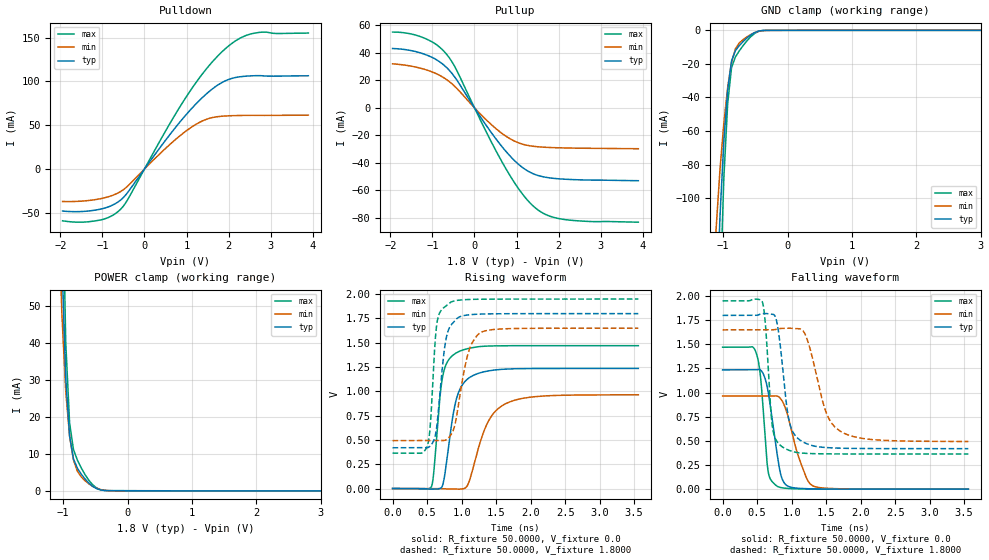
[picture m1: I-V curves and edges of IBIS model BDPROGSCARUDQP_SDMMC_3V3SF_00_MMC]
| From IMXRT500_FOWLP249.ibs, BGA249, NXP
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[Model] BDPROGSCARUDQP_SDMMC_3V3SF_00_MMC
|   Model BDPROGSCARUDQP_SDMMC_3V3SF_00_MMC
| This model was characterised for following simulation conditions:
| External (pad) voltage:
|   - Typ: 1.8V,   - Min: 1.65V,   - Max: 1.95V
| Library cells for typ/min/max conditions are connected as defined below:
|  IO - External Pad
|  A - Core Input
|  EN - Output Buffer Enable
|  ASRCN3V3[0] - REFH3V3
|  ASRCN3V3[1] - REFH3V3
|  ASRCN3V3[2] - REFH3V3
|  ASRCN3V3[3] - REFH3V3
|  ASRCP3V3[0] - REFL3V3
|  ASRCP3V3[1] - REFL3V3
|  ASRCP3V3[2] - REFL3V3
|  ASRCP3V3[3] - REFL3V3
|  IOGC - NC
|  PDRV - gnd
|  PSW - gnd
|  REFH3V3 - REFH3V3
|  REFL3V3 - REFL3V3
|  ZI - NC
|  gnd - gnd
|  gnde - gnde
|  vdd - vdd
|  vdde3v3 - vdde3v3
| All other pins connected to ground
Model_type I/O
Polarity   Non-Inverting
Enable   Active-Low
Vinl =   0.5775V
Vinh =   1.2675V
Vmeas =  0.9000V
Cref =   30.0000pF
Rref =   1.0000M
Vref =   1.8000V
C_comp   2.2202pF   2.2062pF   2.2431pF
|C_comp_pullup   1.1644pF   1.1332pF   1.1986pF
|C_comp_pulldown   0.0F   0.0F   0.0F
[Model Spec]
| variable   typ   min   max
Vinh   1.1700V   1.0725V   1.2675V
Vinl   0.6300V   0.5775V   0.6825V
|[Receiver Thresholds]
[Temperature Range]   25.0000   0.1050k   -20.0000
[Voltage Range]   1.8000V   1.6500V   1.9500V
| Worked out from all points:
|   slope of the pulldown table from 0 to 0.27 V, typ, clamps not added: 15.1 ohm
|   slope of the pullup table from 0 to 0.27 V, typ, clamps not added: 21.9 ohm
|   GND clamp passes 1 mA (typ) near -0.49 V on its own axis
|   POWER clamp passes 1 mA (typ) near -0.52 V on its own axis
|   rising waveform, R_fixture 50.0000, V_fixture 0.0: 20-80 % time 178ps typ, 301ps min, 120ps max; typ from 0 V to 1.24 V
|   rising waveform, R_fixture 50.0000, V_fixture 1.8000: 20-80 % time 121ps typ, 183ps min, 81.3ps max; typ from 0.42 V to 1.8 V
|   falling waveform, R_fixture 50.0000, V_fixture 0.0: 20-80 % time 151ps typ, 232ps min, 93.7ps max; typ from 1.24 V to 0 V
|   falling waveform, R_fixture 50.0000, V_fixture 1.8000: 20-80 % time 138ps typ, 264ps min, 86.9ps max; typ from 1.8 V to 0.42 V
[Pulldown]
|Voltage   I(typ)   I(min)   I(max)
-1.95V    -47.99mA   -37.12mA   -59.11mA
-1.05V    -45.86mA   -33.95mA   -58.21mA
-810mV    -42.31mA   -30.95mA   -54.25mA
-570mV    -35.53mA   -25.76mA   -46.04mA
-390mV    -26.13mA   -19.07mA   -34.15mA
510mV     33.34mA    23.88mA    44.03mA
1.11V     68.35mA    47.41mA    90.64mA
1.65V     92.58mA    59mA       124.1mA
2.07V     103.2mA    60.79mA    142.9mA
2.37V     105.7mA    61.13mA    151.4mA
2.67V     106.5mA    61.18mA    155.4mA
3.9V      106.4mA    61.45mA    155.1mA
[Pullup]
|Voltage   I(typ)   I(min)   I(max)
-1.95V    43.07mA    31.94mA    55mA
-1.2V     39.02mA    28.05mA    50.71mA
-900mV    34.81mA    24.65mA    45.75mA
-660mV    29.15mA    20.42mA    38.73mA
-420mV    20.14mA    14.1mA     27.04mA
240mV     -11.02mA   -7.543mA   -15.06mA
720mV     -30.63mA   -20.03mA   -42.78mA
1.14V     -43.3mA    -26.38mA   -62.56mA
1.5V      -49.04mA   -28.29mA   -73.94mA
1.8V      -50.95mA   -28.84mA   -78.8mA
2.16V     -51.88mA   -29.16mA   -81.21mA
3.9V      -52.96mA   -29.72mA   -83.09mA
[GND_clamp]
|Voltage   I(typ)   I(min)   I(max)
-1.95V    -1.765A    -1.022A    -2.885A
-1.11V    -175mA     -118.7mA   -274.2mA
-1.05V    -111.7mA   -83.43mA   -161.8mA
-990mV    -66.62mA   -55.67mA   -88.75mA
-930mV    -35.53mA   -34.14mA   -43.79mA
-870mV    -18.33mA   -19.05mA   -22.29mA
-810mV    -12.12mA   -11.08mA   -15.87mA
-750mV    -9.12mA    -7.575mA   -12.28mA
-570mV    -2.717mA   -2.477mA   -3.751mA
-450mV    -466.5uA   -625uA     -610.9uA
-330mV    -31.46uA   -57.07uA   -36.76uA
3.9V      0A         0A         0A
[POWER_clamp]
|Voltage   I(typ)   I(min)   I(max)
-1.95V    1.71A      976mA      2.836A
-1.08V    122.1mA    81.01mA    201.9mA
-1.02V    63.03mA    48mA       94.76mA
-960mV    30.4mA     27.02mA    40.25mA
-900mV    14.88mA    14.82mA    18.42mA
-840mV    8.668mA    8.369mA    11.21mA
-780mV    6.192mA    5.372mA    8.379mA
-720mV    4.573mA    3.84mA     6.25mA
-600mV    2.107mA    1.918mA    2.859mA
-480mV    625.6uA    714.7uA    800.1uA
-300mV    67.29uA    79.42uA    85.49uA
3.9V      0A         0A         0A
[Ramp]
| variable   typ   min   max
dV/dt_r  0.7412/0.1778n   0.5784/0.3008n   0.8818/0.1204n
dV/dt_f  0.8278/0.1380n   0.6934/0.2640n   0.9510/86.9648p
R_load = 50.0000
[Rising Waveform]
R_fixture= 50.0000
V_fixture= 0.0
V_fixture_min= 0.0
V_fixture_max= 0.0
|time   V(typ)   V(min)   V(max)
0s        117.6uV    109.5uV    139.1uV
562.4ps   -4.931mV   122.9uV    18.16mV
594.7ps   -4.277mV   173.7uV    152mV
677.9ps   -839.1uV   104.5uV    879.8mV
722.4ps   28.57mV    -1.56mV    1.139V
918ps     903.5mV    -5.529mV   1.394V
1.081ns   1.124V     27.34mV    1.438V
1.376ns   1.209V     676.5mV    1.466V
1.642ns   1.229V     874.3mV    1.469V
3.56ns    1.235V     964mV      1.47V
[Rising Waveform]
R_fixture= 50.0000
V_fixture= 1.8000
V_fixture_min= 1.6500
V_fixture_max= 1.9500
|time   V(typ)   V(min)   V(max)
0s        419.6mV    493.2mV    364.4mV
498.5ps   419.9mV    493.2mV    429.5mV
543.4ps   436.1mV    493.2mV    625mV
614.7ps   533mV      493.3mV    1.496V
647.5ps   681.8mV    493.2mV    1.722V
753.3ps   1.446V     495.5mV    1.868V
838.5ps   1.672V     545.1mV    1.915V
1.093ns   1.786V     1.388V     1.945V
1.264ns   1.795V     1.6V       1.948V
3.56ns    1.799V     1.649V     1.949V
[Falling Waveform]
R_fixture= 50.0000
V_fixture= 0.0
V_fixture_min= 0.0
V_fixture_max= 0.0
|time   V(typ)   V(min)   V(max)
0s        1.235V     964mV      1.47V
479.1ps   1.236V     964.3mV    1.426V
549.2ps   1.234V     964.2mV    1.168V
660.6ps   1.008V     964mV      181.4mV
790.5ps   364mV      964.1mV    30.51mV
847.8ps   138.2mV    931.1mV    16.13mV
916ps     45.91mV    827.4mV    9.318mV
1.116ns   8.351mV    304mV      2.793mV
1.315ns   3.043mV    32.47mV    1.081mV
3.56ns    124.6uV    222.5uV    139.7uV
[Falling Waveform]
R_fixture= 50.0000
V_fixture= 1.8000
V_fixture_min= 1.6500
V_fixture_max= 1.9500
|time   V(typ)   V(min)   V(max)
0s        1.799V     1.649V     1.949V
574.9ps   1.816V     1.649V     1.942V
622.1ps   1.819V     1.649V     1.695V
721.6ps   1.812V     1.65V      648.1mV
797.2ps   1.688V     1.659V     484.2mV
886.8ps   1.141V     1.666V     428.2mV
964.9ps   704.2mV    1.667V     401.9mV
1.057ns   550.6mV    1.663V     381.9mV
1.717ns   424.1mV    595.4mV    364.6mV
3.56ns    419.6mV    493.7mV    364.3mV
